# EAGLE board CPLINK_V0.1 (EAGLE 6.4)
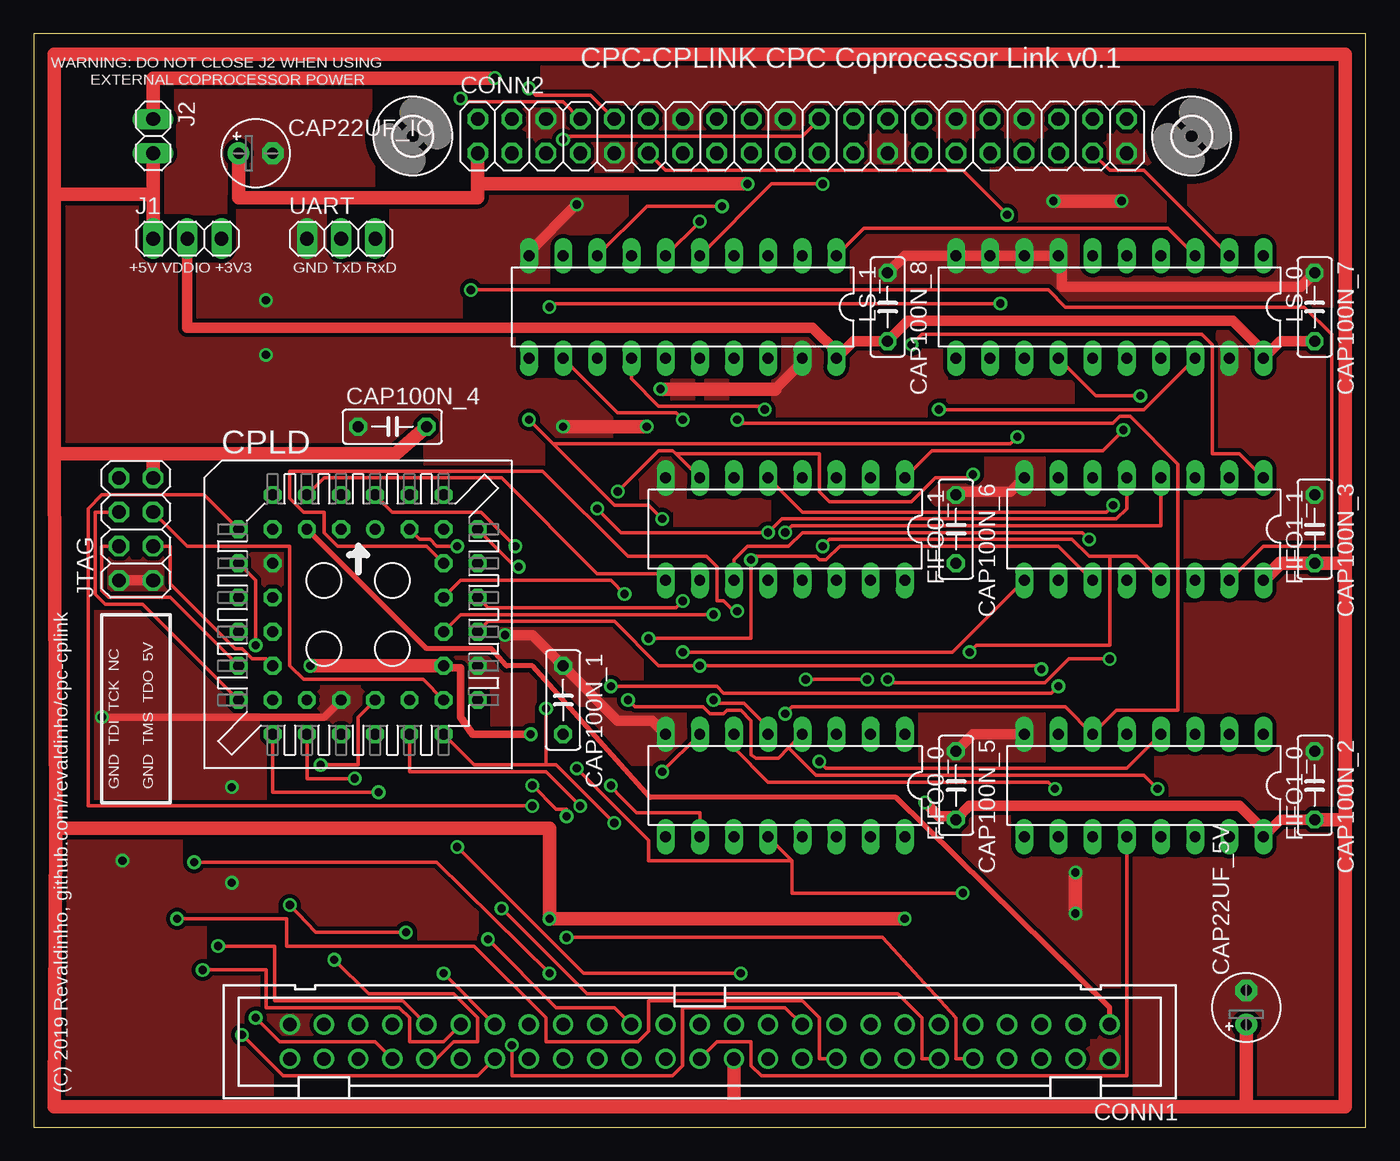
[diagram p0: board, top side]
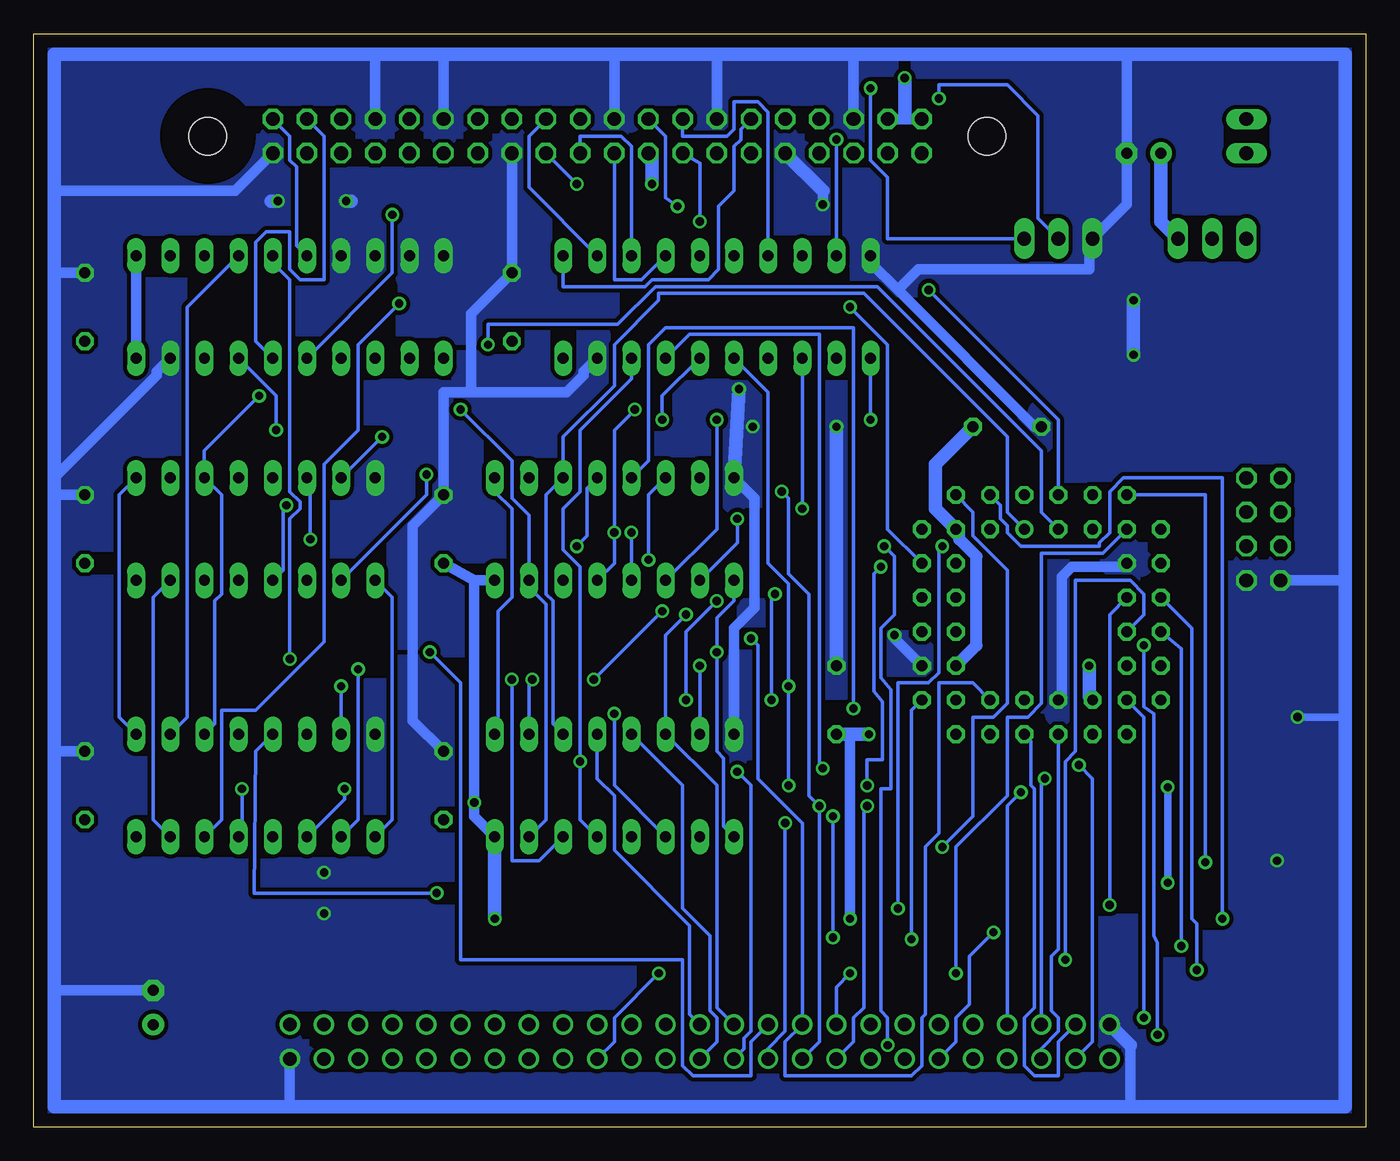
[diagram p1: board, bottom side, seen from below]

Size 99.06 x 81.28 mm. Coordinates in mm from the lower left corner, seen from the top.
Outline: 0,0 99.06,0 99.06,81.28 0,81.28 0,0
Copper layers (1*16): Top 0.035mm / dielectric 1.5mm / Bottom 0.035mm
Design rules "default": minimum track width 10mil, minimum drill 24mil, track to track 8mil, track to pad 8mil, pad to pad 8mil, via to via 8mil, smd to smd 8mil, copper to edge 40mil, drill to drill 8mil, minimum pad ring 10mil, minimum via ring 8mil, stop-mask expansion 4mil, vias tented up to drill 0mil, thermal gap 10mil
Net classes: 0 signal: width 0.254 mm, clearance 0.254 mm; 1 supply: width 0.559 mm, clearance 0.305 mm

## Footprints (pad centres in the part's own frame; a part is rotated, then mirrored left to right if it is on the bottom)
E2,5-5 = drill 0.813 pad 1.6: + -1.27,0 | drill 0.813 pad 1.6 octagon: - 1.27,0
C050-025X075 = drill 0.813 octagon: 1 -2.54,0; 2 2.54,0
PAK100/2500-50 = drill 1 pad 1.422: 1 -30.48,-1.27; 2 -30.48,1.27; 3 -27.94,-1.27; 4 -27.94,1.27; 5 -25.4,-1.27; 6 -25.4,1.27; 7 -22.86,-1.27; 8 -22.86,1.27; 9 -20.32,-1.27; 10 -20.32,1.27; 11 -17.78,-1.27; 12 -17.78,1.27; 13 -15.24,-1.27; 14 -15.24,1.27; 15 -12.7,-1.27; 16 -12.7,1.27; 17 -10.16,-1.27; 18 -10.16,1.27; 19 -7.62,-1.27; 20 -7.62,1.27; 21 -5.08,-1.27; 22 -5.08,1.27; 23 -2.54,-1.27; 24 -2.54,1.27; 25 0,-1.27; 26 0,1.27; 27 2.54,-1.27; 28 2.54,1.27; 29 5.08,-1.27; 30 5.08,1.27; 31 7.62,-1.27; 32 7.62,1.27; 33 10.16,-1.27; 34 10.16,1.27; 35 12.7,-1.27; 36 12.7,1.27; 37 15.24,-1.27; 38 15.24,1.27; 39 17.78,-1.27; 40 17.78,1.27; 41 20.32,-1.27; 42 20.32,1.27; 43 22.86,-1.27; 44 22.86,1.27; 45 25.4,-1.27; 46 25.4,1.27; 47 27.94,-1.27; 48 27.94,1.27; 49 30.48,-1.27; 50 30.48,1.27
2X20 = drill 1.016 octagon: 1 -24.13,-1.27; 2 -24.13,1.27; 3 -21.59,-1.27; 4 -21.59,1.27; 5 -19.05,-1.27; 6 -19.05,1.27; 7 -16.51,-1.27; 8 -16.51,1.27; 9 -13.97,-1.27; 10 -13.97,1.27; 11 -11.43,-1.27; 12 -11.43,1.27; 13 -8.89,-1.27; 14 -8.89,1.27; 15 -6.35,-1.27; 16 -6.35,1.27; 17 -3.81,-1.27; 18 -3.81,1.27; 19 -1.27,-1.27; 20 -1.27,1.27; 21 1.27,-1.27; 22 1.27,1.27; 23 3.81,-1.27; 24 3.81,1.27; 25 6.35,-1.27; 26 6.35,1.27; 27 8.89,-1.27; 28 8.89,1.27; 29 11.43,-1.27; 30 11.43,1.27; 31 13.97,-1.27; 32 13.97,1.27; 33 16.51,-1.27; 34 16.51,1.27; 35 19.05,-1.27; 36 19.05,1.27; 37 21.59,-1.27; 38 21.59,1.27; 39 24.13,-1.27; 40 24.13,1.27
PLCC-S44-SOCKET = drill 0.813: 1 1.27,6.35 | drill 0.813 octagon: 2 -1.27,8.89; 3 -1.27,6.35; 4 -3.81,8.89; 5 -3.81,6.35; 6 -6.35,8.89; 7 -8.89,6.35; 8 -6.35,6.35; 9 -8.89,3.81; 10 -6.35,3.81; 11 -8.89,1.27; 12 -6.35,1.27; 13 -8.89,-1.27; 14 -6.35,-1.27; 15 -8.89,-3.81; 16 -6.35,-3.81; 17 -8.89,-6.35; 18 -6.35,-8.89; 19 -6.35,-6.35; 20 -3.81,-8.89; 21 -3.81,-6.35; 22 -1.27,-8.89; 23 -1.27,-6.35; 24 1.27,-8.89; 25 1.27,-6.35; 26 3.81,-8.89; 27 3.81,-6.35; 28 6.35,-8.89; 29 8.89,-6.35; 30 6.35,-6.35; 31 8.89,-3.81; 32 6.35,-3.81; 33 8.89,-1.27; 34 6.35,-1.27; 35 8.89,1.27; 36 6.35,1.27; 37 8.89,3.81; 38 6.35,3.81; 39 8.89,6.35; 40 6.35,8.89; 41 6.35,6.35; 42 3.81,8.89; 43 3.81,6.35; 44 1.27,8.89
DIL16 = drill 0.813 long: 1 -8.89,-3.81; 2 -6.35,-3.81; 3 -3.81,-3.81; 4 -1.27,-3.81; 5 1.27,-3.81; 6 3.81,-3.81; 7 6.35,-3.81; 8 8.89,-3.81; 9 8.89,3.81; 10 6.35,3.81; 11 3.81,3.81; 12 1.27,3.81; 13 -1.27,3.81; 14 -3.81,3.81; 15 -6.35,3.81; 16 -8.89,3.81
2,8 = hole 2.8: 0,0
1X03 = drill 1.016 long: 1 -2.54,0; 2 0,0; 3 2.54,0
1X02 = drill 1.016 long: 1 -1.27,0; 2 1.27,0
2X04 = drill 1.016 octagon: 1 -3.81,-1.27; 2 -3.81,1.27; 3 -1.27,-1.27; 4 -1.27,1.27; 5 1.27,-1.27; 6 1.27,1.27; 7 3.81,-1.27; 8 3.81,1.27
DIL20 = drill 0.813 long: 1 -11.43,-3.81; 2 -8.89,-3.81; 3 -6.35,-3.81; 4 -3.81,-3.81; 5 -1.27,-3.81; 6 1.27,-3.81; 7 3.81,-3.81; 8 6.35,-3.81; 9 8.89,-3.81; 10 11.43,-3.81; 11 11.43,3.81; 12 8.89,3.81; 13 6.35,3.81; 14 3.81,3.81; 15 1.27,3.81; 16 -1.27,3.81; 17 -3.81,3.81; 18 -6.35,3.81; 19 -8.89,3.81; 20 -11.43,3.81

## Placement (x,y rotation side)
CAP22UF_5V  [E2,5-5]  90.17,8.89 90 top
CAP22UF_IO  [E2,5-5]  16.51,72.39 0 top
CAP100N_1  [C050-025X075]  39.37,31.75 270 top
CAP100N_2  [C050-025X075]  95.25,25.4 270 top
CAP100N_3  [C050-025X075]  95.25,44.45 270 top
CAP100N_4  [C050-025X075]  26.67,52.07 0 top
CAP100N_5  [C050-025X075]  68.58,25.4 270 top
CAP100N_6  [C050-025X075]  68.58,44.45 270 top
CAP100N_7  [C050-025X075]  95.25,60.96 270 top
CAP100N_8  [C050-025X075]  63.5,60.96 270 top
CONN1  [PAK100/2500-50]  49.53,6.35 180 top
CONN2  [2X20]  57.15,73.66 0 top
CPLD  [PLCC-S44-SOCKET]  24.13,38.1 0 top
FIFO0_0  [DIL16]  55.88,25.4 180 top
FIFO0_1  [DIL16]  55.88,44.45 180 top
FIFO1_0  [DIL16]  82.55,25.4 180 top
FIFO1_1  [DIL16]  82.55,44.45 180 top
H1  [2,8]  86.11,73.66 0 top
H2  [2,8]  28.19,73.66 0 top
J1  [1X03]  11.43,66.04 0 top
J2  [1X02]  8.89,73.66 270 top
JTAG  [2X04]  7.62,44.45 90 top
LS_0  [DIL20]  80.01,60.96 180 top
LS_1  [DIL20]  48.26,60.96 180 top
UART  [1X03]  22.86,66.04 0 top

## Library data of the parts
CAP22UF_5V CAP22UF_IO CAP100N_1-CAP100N_8 = resistor
CONN1 = con-3m
CONN2 J1 J2 JTAG UART = pinhead
CPLD FIFO0_0 FIFO0_1 FIFO1_0 FIFO1_1 LS_0 LS_1 = ic-package
H1 H2 = holes

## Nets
A0: CONN1.33 CPLD.6
A1: CONN1.34 CPLD.7
A2: CONN1.35
A3: CONN1.36
A4: CONN1.37 CPLD.8
A5: CONN1.38 CPLD.9
A6: CONN1.39 CPLD.11
A7: CONN1.40 CPLD.12
A8: CONN1.41 CPLD.13
A9: CONN1.42 CPLD.14
A10: CONN1.43 CPLD.18
A11: CONN1.44 CPLD.19
A12: CONN1.45 CPLD.20
A13: CONN1.46 CPLD.22
A14: CONN1.47 CPLD.24
A15: CONN1.48 CPLD.25
BUSACK_B: CONN1.13
BUSRESET_B: CONN1.11
BUSRQ_B: CONN1.14
CLK: CONN1.1 CPLD.5
CURSOR: CONN1.5
D0: CONN1.25 CPLD.36 FIFO0_0.4 FIFO1_0.13
D1: CONN1.26 CPLD.35 FIFO0_0.5 FIFO1_0.12
D2: CONN1.27 CPLD.34 FIFO0_0.6 FIFO1_0.11
D3: CONN1.28 CPLD.33 FIFO0_0.7 FIFO1_0.10
D4: CONN1.29 CPLD.29 FIFO0_1.4 FIFO1_1.13
D5: CONN1.30 CPLD.28 FIFO0_1.5 FIFO1_1.12
D6: CONN1.31 CPLD.27 FIFO0_1.6 FIFO1_1.11
D7: CONN1.32 CPLD.26 FIFO0_1.7 FIFO1_1.10
EXP_B: CONN1.3
FIFO_HOST_DIR: CPLD.38 FIFO0_0.2
FIFO_HOST_DOR: CPLD.37 FIFO1_0.14
FIFO_SLAVE_DIR: FIFO1_0.2 LS_0.4
FIFO_SLAVE_DOR: FIFO0_0.14 LS_0.5
HALT_B: CONN1.17
HOST_FIFO_OEB: CPLD.3 FIFO1_0.1 FIFO1_1.1
HOST_FIFO_RESET: CPLD.4 FIFO0_0.9 FIFO0_1.9 FIFO1_0.9 FIFO1_1.9
HOST_FIFO_SI: CPLD.1 FIFO0_0.3 FIFO0_1.3
HOST_FIFO_SOB: CPLD.2 FIFO1_0.15 FIFO1_1.15
INT_B: CONN1.16
IOREQ_B: CONN1.20 CPLD.40
LPEN: CONN1.4
M1_B: CONN1.22
MREQ_B: CONN1.23
NMI_B: CONN1.15
PI_GPIO_02: CONN2.3
PI_GPIO_03: CONN2.5
PI_GPIO_04: CONN2.7
PI_GPIO_05: CONN2.29
PI_GPIO_06: CONN2.31
PI_GPIO_07: CONN2.26
PI_GPIO_08: CONN2.24 LS_1.2
PI_GPIO_09: CONN2.21 LS_1.3
PI_GPIO_10: CONN2.19 LS_1.4
PI_GPIO_11: CONN2.23 LS_1.5
PI_GPIO_12: CONN2.32
PI_GPIO_13: CONN2.33
PI_GPIO_14: CONN2.8 UART.2
PI_GPIO_15: CONN2.10 UART.3
PI_GPIO_16: CONN2.36
PI_GPIO_17: CONN2.11 LS_0.15
PI_GPIO_18: CONN2.12 LS_0.3 LS_1.1
PI_GPIO_19: CONN2.35
PI_GPIO_20: CONN2.38 LS_0.16
PI_GPIO_21: CONN2.40 LS_0.6
PI_GPIO_22: CONN2.15 LS_1.6
PI_GPIO_23: CONN2.16 LS_1.7
PI_GPIO_24: CONN2.18 LS_1.8
PI_GPIO_25: CONN2.22 LS_1.9
PI_GPIO_26: CONN2.37 LS_0.2
PI_GPIO_27: CONN2.13
RAMDIS: CONN1.6
RAMRD_B: CONN1.7
RD_B: CONN1.19 CPLD.44
READY: CONN1.12 CPLD.43
RESET_B: CONN1.10 CPLD.39
RFSH_B: CONN1.21
ROMDIS: CONN1.8
ROMEN_B: CONN1.9
SCL: CONN2.28
SD0: FIFO0_0.13 FIFO1_0.4 LS_1.18
SD1: FIFO0_0.12 FIFO1_0.5 LS_1.17
SD2: FIFO0_0.11 FIFO1_0.6 LS_1.16
SD3: FIFO0_0.10 FIFO1_0.7 LS_1.15
SD4: FIFO0_1.13 FIFO1_1.4 LS_1.14
SD5: FIFO0_1.12 FIFO1_1.5 LS_1.13
SD6: FIFO0_1.11 FIFO1_1.6 LS_1.12
SD7: FIFO0_1.10 FIFO1_1.7 LS_1.11
SDA: CONN2.27
SLAVE_FIFO_SI: FIFO1_0.3 FIFO1_1.3 LS_0.14
SLAVE_FIFO_SOB: FIFO0_0.15 FIFO0_1.15 LS_0.18
SLAVE_FIFO_WNR: FIFO0_0.1 FIFO0_1.1 LS_0.17
SOUND: CONN1.50
TCK: CPLD.17 JTAG.6
TDI: CPLD.15 JTAG.4
TDO: CPLD.30 JTAG.5
TMS: CPLD.16 JTAG.3
VDD [supply]: CAP22UF_5V.+ CAP100N_1.2 CAP100N_2.2 CAP100N_3.2 CAP100N_4.2 CAP100N_5.2 CAP100N_6.2 CONN1.24 CPLD.21 CPLD.32 CPLD.41 FIFO0_0.16 FIFO0_1.16 FIFO1_0.16 FIFO1_1.16 J1.1 J2.2 JTAG.7
VDD_3V3 [supply]: CAP22UF_IO.+ CONN2.1 CONN2.17 J1.3
VDD_IO [supply]: CAP100N_7.2 CAP100N_8.2 J1.2 LS_0.1 LS_0.20 LS_1.20
VDD_PI [supply]: CONN2.2 CONN2.4 J2.1
VSS [supply]: CAP22UF_5V.- CAP22UF_IO.- CAP100N_1.1 CAP100N_2.1 CAP100N_3.1 CAP100N_4.1 CAP100N_5.1 CAP100N_6.1 CAP100N_7.1 CAP100N_8.1 CONN1.2 CONN1.49 CONN2.6 CONN2.9 CONN2.14 CONN2.20 CONN2.25 CONN2.30 CONN2.34 CONN2.39 CPLD.10 CPLD.23 CPLD.31 FIFO0_0.8 FIFO0_1.8 FIFO1_0.8 FIFO1_1.8 JTAG.1 JTAG.2 LS_0.7 LS_0.8 LS_0.9 LS_0.10 LS_0.19 LS_1.10 LS_1.19 UART.1
WR_B: CONN1.18 CPLD.42

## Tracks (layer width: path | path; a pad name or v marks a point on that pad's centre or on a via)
A0  (via drill 0.61)
  Top 0.254: v11.94,19.68 29.97,19.68 v38.35,11.43
  Bottom 0.254: CPLD.6 11.94,46.99 v11.94,19.68 | v38.35,11.43 39.37,10.41 CONN1.33
A1  (via drill 0.61)
  Top 0.254: CPLD.7 12.7,46.99 5.08,46.99 4.06,45.97 4.06,23.88 v37.08,23.88
  Bottom 0.254: v37.08,23.88 37.34,23.62 37.34,8.89 38.1,8.13 38.1,6.35 CONN1.34
A4  (via drill 0.61)
  Top 0.254: CONN1.37 v30.48,11.43
  Bottom 0.254: CPLD.8 19.56,42.67 24.13,42.67 24.13,31.5 25.15,30.48 26.67,30.48 26.67,24.64 30.48,20.83 v30.48,11.43
A5  (via drill 0.61)
  Top 0.254: CPLD.9 16.51,40.64 v16.51,35.81 | v15.49,6.86 18.54,3.81 33.02,3.81 CONN1.38
  Bottom 0.254: v16.51,35.81 16.51,31.24 15.75,30.73 15.75,14.22 15.49,13.72 v15.49,6.86
A6  (via drill 0.61)
  Top 0.254: v12.57,11.68 17.27,11.68 17.27,8.89 27.18,8.89 27.94,8.13 27.94,6.35 30.48,6.35 CONN1.39
  Bottom 0.254: CPLD.11 12.95,37.08 12.95,15.49 12.57,15.11 v12.57,11.68
A7  (via drill 0.61)
  Top 0.254: v27.69,14.48 20.95,14.48 19.68,15.88 v19.05,16.51
  Bottom 0.254: CPLD.12 19.05,38.1 v19.05,16.51 | v27.69,14.48 29.46,12.7 29.46,9.14 30.48,8.13 30.48,6.35 CONN1.40
A8  (via drill 0.61)
  Top 0.254: v13.72,13.46 17.91,13.46 17.91,9.4 27.43,9.4 CONN1.41
  Bottom 0.254: CPLD.13 13.72,35.56 v13.72,13.46
A9  (via drill 0.61)
  Top 0.254: v22.35,12.45 24.89,9.91 31.24,9.91 33.02,8.13 33.02,6.35 31.24,6.35 29.97,5.08 CONN1.42
  Bottom 0.254: CPLD.14 16.51,38.1 16.51,39.62 17.53,40.64 21.59,40.64 21.59,27.94 22.35,27.18 v22.35,12.45
A10  (via drill 0.61)
  Top 0.254: CPLD.18 17.78,24.89 v25.65,24.89
  Bottom 0.254: v25.65,24.89 26.67,23.88 CONN1.43
A11  (via drill 0.61)
  Top 0.254: v16.51,8.13 18.29,6.35 25.4,6.35 CONN1.44
  Bottom 0.254: CPLD.19 16.51,30.48 v16.51,8.13
A12  (via drill 0.61)
  Top 0.254: CPLD.20 20.32,25.91 v23.88,25.91
  Bottom 0.254: v23.88,25.91 24.13,25.65 CONN1.45
A13
  Bottom 0.254: CPLD.22 22.86,13.21 23.37,12.7 23.37,8.64 22.86,8.13 22.86,7.11 24.13,5.84 CONN1.46
A14
  Bottom 0.254: CPLD.24 24.89,28.7 24.89,25.4 24.64,25.15 24.64,8.89 25.4,8.13 25.4,4.57 24.64,3.81 22.86,3.81 22.86,6.35 CONN1.47
A15  (via drill 0.61)
  Top 0.254: CPLD.25 24.13,30.48 24.13,26.92 v21.34,26.92
  Bottom 0.254: v21.34,26.92 20.32,25.91 20.32,6.35 CONN1.48
CLK
  Top 0.381: CPLD.5 29.21,35.56 34.04,35.56 35.18,34.29 37.08,34.29 45.85,24.51 64.14,24.51 80.01,8.89 CONN1.1
D0  (via drill 0.61)
  Top 0.254: CPLD.36 31.75,40.64 42.93,40.64 v43.94,39.62 | v44.2,31.75 44.7,31.24 49.78,31.24 50.29,30.73 51.31,30.73 51.56,30.99 52.58,30.99 53.34,30.23 53.34,27.69 53.72,27.43 55.37,27.43 56.13,28.19 | FIFO0_0.4 56.13,28.19 | v83.57,25.15 82.55,26.16 58.17,26.16 56.13,28.19
  Bottom 0.254: v43.94,39.62 44.2,39.37 v44.2,31.75 | FIFO1_0.13 83.57,21.84 v83.57,25.15 | CONN1.25 50.29,8.38 50.29,14.99 55.88,20.57 55.88,24.64 57.15,25.91 FIFO0_0.4
D1  (via drill 0.61)
  Top 0.254: FIFO1_0.12 81.28,3.81 54.1,3.81 53.34,4.57 53.34,6.35 50.8,6.35 CONN1.26 | CPLD.35 33.78,38.61 47.75,38.61 v48.26,39.12 | v50.55,31.75 50.8,31.5 52.83,31.5 54.61,29.72 FIFO0_0.5
  Bottom 0.254: FIFO0_0.5 50.8,25.4 50.8,16.26 48.77,14.22 48.77,8.64 48.26,8.13 48.26,6.35 CONN1.26 | v48.26,39.12 50.55,36.83 v50.55,31.75
D2  (via drill 0.61)
  Top 0.254: CPLD.34 31.75,38.1 v50.55,38.1 | v75.95,25.15 75.44,25.65 54.61,25.65 52.07,28.19 FIFO0_0.6
  Bottom 0.254: v50.55,38.1 52.07,36.58 FIFO0_0.6 48.26,25.4 48.26,8.89 CONN1.27 | FIFO1_0.11 75.95,24.38 v75.95,25.15
D3  (via drill 0.61)
  Top 0.254: CPLD.33 33.78,37.59 43.18,37.59 46.48,34.29 v49.53,34.29 74.68,34.29 v74.93,34.04 | FIFO0_0.7 v46.74,26.42
  Bottom 0.254: FIFO0_0.7 v49.53,34.29 | FIFO1_0.10 74.93,22.86 v74.93,34.04 | CONN1.28 46.23,5.84 46.23,6.6 45.72,7.11 45.72,25.4 v46.74,26.42
D4  (via drill 0.61)
  Top 0.254: v58.67,43.18 59.18,43.69 77.22,43.69 78.49,42.42 80.01,42.42 | 80.01,42.42 82.04,42.42 FIFO1_1.13 | v33.78,13.97 38.86,8.89 43.18,8.89 CONN1.29 | 80.01,42.42 80.01,35.81 70.1,35.81 v69.6,35.31
  Bottom 0.254: FIFO0_1.4 57.91,47.5 57.91,43.94 v58.67,43.18 | CPLD.29 33.78,30.99 v33.78,13.97 | v69.6,35.31 67.31,33.02 67.31,12.45 50.8,12.45 50.8,4.57 50.04,3.81 45.72,3.81 45.72,6.35 CONN1.29
D5  (via drill 0.61)
  Top 0.254: v80.26,46.23 79.76,45.72 57.15,45.72 FIFO0_1.5 | CPLD.28 32.77,26.92 38.1,26.92 | 38.1,26.92 38.86,26.92 v43.18,22.61 | 38.1,26.92 v38.1,31.11
  Bottom 0.254: FIFO1_1.12 80.52,41.4 80.52,45.97 v80.26,46.23 | v43.18,22.61 43.18,7.11 44.45,5.84 CONN1.30 | FIFO0_1.5 53.34,49.53 53.34,58.17 52.07,59.44 38.1,59.44 v38.1,31.11
D6  (via drill 0.61)
  Top 0.254: FIFO1_1.11 76.2,43.18 59.94,43.18 58.93,42.16 58.42,42.16 58.17,42.42 53.59,42.42 v53.34,42.16 53.34,36.32 v45.72,36.32
  Bottom 0.254: FIFO0_1.6 53.34,46.99 v53.34,42.16 | CPLD.27 29.21,33.02 31.75,33.02 31.75,21.84 32.77,20.83 32.77,8.38 33.02,8.13 33.02,4.57 33.78,3.81 43.18,3.81 43.18,6.35 CONN1.31 41.91,22.61 45.21,25.91 45.21,35.81 v45.72,36.32
D7  (via drill 0.61)
  Top 0.254: CPLD.26 27.94,26.42 38.1,26.42 v40.64,23.88 | 47.75,50.04 47.5,50.29 46.48,50.29 v43.43,47.24 | 47.75,50.04 FIFO0_1.7 | v69.85,48.51 69.6,48.26 67.06,48.26 65.28,46.48 59.18,46.48 58.42,47.24 58.42,50.04 47.75,50.04
  Bottom 0.254: CONN1.32 40.64,6.35 v40.64,23.88 41.4,24.64 41.4,39.62 42.93,41.15 42.93,46.74 v43.43,47.24 | FIFO1_1.10 69.85,46.99 v69.85,48.51
FIFO_HOST_DIR  (via drill 0.61)
  Top 0.254: CPLD.38 29.21,43.18 22.61,43.18 21.59,44.2 21.59,45.72 20.07,45.72 19.05,46.74 19.05,48.77 37.85,48.77 44.2,42.42 50.04,42.42 50.8,41.66 50.8,39.12 51.31,39.12 52.07,38.35 v52.32,38.35 | v61.98,33.27 v57.4,33.27
  Bottom 0.254: v57.4,33.27 v52.32,38.35 | v61.98,33.27 62.23,33.02 FIFO0_0.2
FIFO_HOST_DOR  (via drill 0.61)
  Top 0.254: v38.35,60.96 38.61,61.21 v71.88,61.21
  Bottom 0.254: CPLD.37 35.56,44.45 35.56,58.17 v38.35,60.96 | v71.88,61.21 74.93,58.17 74.93,51.82 77.47,49.28 77.47,36.07 82.55,30.99 85.09,30.99 85.09,22.86 FIFO1_0.14
FIFO_SLAVE_DIR
  Bottom 0.254: FIFO1_0.2 87.63,30.48 87.63,60.96 LS_0.4
FIFO_SLAVE_DOR  (via drill 0.61)
  Top 0.254: v63.5,33.27 63.75,33.02 75.18,33.02 76.96,34.8 v80.01,34.8
  Bottom 0.254: FIFO0_0.14 61.47,19.81 63.5,19.81 v63.5,33.27 | v80.01,34.8 80.01,45.21 79.25,45.97 79.25,46.48 80.01,47.24 80.01,62.99 81.28,64.26 LS_0.5
HOST_FIFO_OEB  (via drill 0.61)
  Top 0.254: v65.28,58.17 66.04,58.93 86.87,58.93 87.63,58.17 87.63,50.04 89.66,50.04 FIFO1_1.1
  Bottom 0.254: CPLD.3 24.13,45.72 24.13,50.29 36.32,62.48 52.83,62.48 55.63,59.69 65.28,59.69 v65.28,58.17 | FIFO1_0.1 92.71,30.48 92.71,46.99 FIFO1_1.1
HOST_FIFO_RESET  (via drill 0.61)
  Top 0.254: CPLD.4 21.59,48.26 34.8,48.26 41.91,41.15 46.48,41.15 FIFO0_1.9 | FIFO1_1.9 68.33,35.31 v48.26,35.31
  Bottom 0.254: FIFO1_0.9 72.39,22.86 72.39,39.37 FIFO1_1.9 | FIFO0_0.9 47.75,22.35 47.75,27.43 48.26,27.94 v48.26,35.31 48.26,37.85 46.99,39.12 FIFO0_1.9
HOST_FIFO_SI
  Bottom 0.254: CPLD.1 26.67,45.72 26.67,51.31 37.34,61.98 52.58,61.98 52.58,61.47 55.88,58.17 55.88,55.12 59.69,51.31 FIFO0_1.3 60.96,46.99 60.96,39.62 60.45,39.12 60.45,29.97 FIFO0_0.3
HOST_FIFO_SOB  (via drill 0.61)
  Top 0.254: v32.51,62.23 75.44,62.23 76.71,60.96 94.49,60.96 96.52,58.93 96.52,43.18 91.44,43.18 FIFO1_1.15
  Bottom 0.254: FIFO1_0.15 90.17,22.86 90.17,39.37 FIFO1_1.15 | CPLD.2 22.86,52.58 v32.51,62.23
IOREQ_B  (via drill 0.61)
  Top 0.254: v31.5,20.83 40.89,11.43 v52.58,11.43
  Bottom 0.254: CPLD.40 29.21,45.72 29.21,43.94 26.67,41.4 26.67,31.5 27.69,30.48 29.21,30.48 29.21,23.11 v31.5,20.83 | v52.58,11.43 55.88,8.13 55.88,6.35 CONN1.20
PI_GPIO_08
  Bottom 0.254: LS_1.2 62.23,69.85 62.23,73.66 CONN2.24
PI_GPIO_09
  Bottom 0.254: LS_1.3 54.61,72.9 55.37,73.66 58.42,73.66 CONN2.21
PI_GPIO_10
  Bottom 0.254: LS_1.4 53.85,62.99 55.88,62.99 CONN2.19
PI_GPIO_11  (via drill 0.61)
  Top 0.254: LS_1.5 54.86,70.1 v58.67,70.1
  Bottom 0.254: CONN2.23 v58.67,70.1
PI_GPIO_14  (via drill 0.61)
  Top 0.254: v31.75,76.45 32,76.2 39.37,76.2 CONN2.8
  Bottom 0.254: UART.2 24.38,67.56 24.38,75.18 26.67,77.47 31.75,77.47 v31.75,76.45
PI_GPIO_15  (via drill 0.61)
  Top 0.254: v36.83,77.22 37.34,76.71 41.4,76.71 CONN2.10
  Bottom 0.254: UART.3 35.56,66.04 35.56,70.61 36.83,71.88 v36.83,77.22
PI_GPIO_17  (via drill 0.61)
  Top 0.254: v72.39,67.82 69.09,71.12 46.99,71.12 CONN2.11
  Bottom 0.254: LS_0.15 72.39,63.5 v72.39,67.82
PI_GPIO_18
  Top 0.254: LS_1.1 61.72,66.8 84.33,66.8 LS_0.3
  Bottom 0.254: CONN2.12 46.48,74.17 46.48,73.41 46.99,72.9 46.99,69.6 48.13,68.45 48.13,63.75 48.9,62.99 53.09,62.99 53.59,62.48 59.69,62.48 LS_1.1
PI_GPIO_20
  Bottom 0.254: LS_0.16 82.55,58.42 82.55,65.79 81.79,66.55 80.01,66.55 80.01,63.75 79.25,62.99 77.47,62.99 77.47,73.66 CONN2.38
PI_GPIO_21
  Bottom 0.254: LS_0.6 79.5,65.53 79.5,71.37 80.01,71.88 80.01,73.66 CONN2.40
PI_GPIO_22  (via drill 0.61)
  Top 0.254: v49.53,67.31 LS_1.6
  Bottom 0.254: v49.53,67.31 49.53,71.63 CONN2.15
PI_GPIO_23
  Bottom 0.254: LS_1.7 44.45,75.44 45.21,76.2 46.99,76.2 46.99,74.17 47.5,73.66 50.8,73.66 CONN2.16
PI_GPIO_24  (via drill 0.61)
  Top 0.254: LS_1.8 45.59,68.45 v51.18,68.45
  Bottom 0.254: v51.18,68.45 52.07,69.09 52.07,73.66 CONN2.18
PI_GPIO_25  (via drill 0.61)
  Top 0.254: v39.37,73.41 39.62,73.66 57.15,73.66 CONN2.22
  Bottom 0.254: v39.37,73.41 LS_1.9
PI_GPIO_26
  Top 0.254: LS_0.2 82.55,71.12 80.01,71.12 CONN2.37
RD_B  (via drill 0.61)
  Top 0.254: CPLD.44 26.67,45.72 33.27,45.72 v35.81,43.18 | v35.56,6.1 35.56,3.81 47.5,3.81 48.26,4.57 48.26,8.89 55.88,8.89 CONN1.19
  Bottom 0.254: v35.81,43.18 35.05,42.42 35.05,38.1 36.07,37.08 36.07,33.4 35.31,32.51 35.31,25.15 36.07,25.15 36.07,8.64 35.56,8.13 v35.56,6.1
READY  (via drill 0.61)
  Top 0.254: CPLD.43 28.7,43.69 29.46,43.69 29.97,43.18 v31.5,43.18 | v34.8,16.26 41.15,9.91 64.26,9.91 66.04,8.13 66.04,5.08 CONN1.12
  Bottom 0.254: v31.5,43.18 31.75,42.93 31.75,33.78 32.51,33.02 34.8,33.02 v34.8,16.26
RESET_B  (via drill 0.61)
  Top 0.254: CPLD.39 35.81,41.66 v36.07,41.66 | v37.08,25.4 38.86,23.62 39.62,23.62 v39.62,23.11 | v39.62,14.1 63.12,14.1 68.58,8.13 68.58,5.08 CONN1.10
  Bottom 0.254: v36.07,41.66 36.58,41.15 36.58,32.38 35.94,31.62 35.94,27.3 37.08,27.3 v37.08,25.4 | v39.62,14.1 v39.62,23.11
SD0  (via drill 0.61)
  Top 0.254: FIFO1_0.4 81.28,26.67 58.93,26.67 v58.42,27.18
  Bottom 0.254: FIFO0_0.13 58.42,22.86 v58.42,27.18 58.42,41.66 59.69,42.93 59.69,45.97 58.42,47.24 58.42,51.82 54.61,55.63 LS_1.18
SD1  (via drill 0.61)
  Top 0.254: 56.39,19.81 56.39,17.4 v69.09,17.4 | 56.39,19.81 FIFO0_0.12 | v40.39,26.67 45.72,21.34 45.72,19.81 56.39,19.81
  Bottom 0.254: v69.09,17.4 82.68,17.4 82.55,27.94 FIFO1_0.5 | LS_1.17 50.29,58.93 40.64,58.93 40.64,26.92 v40.39,26.67
SD2  (via drill 0.61)
  Top 0.254: v55.88,30.73 56.39,31.24 76.71,31.24 FIFO1_0.6 80.52,30.99 85.09,30.99 85.09,49.28 81.53,52.83 80.77,52.83 80.26,52.32 52.58,52.32 v52.32,52.58
  Bottom 0.254: FIFO0_0.11 55.88,25.4 v55.88,30.73 | LS_1.16 52.32,54.36 v52.32,52.58
SD3  (via drill 0.61)
  Top 0.254: FIFO0_0.10 49.53,23.37 44.83,23.37 43.43,24.77 v42.93,25.4 | v76.2,32.77 75.69,32.26 51.31,32.26 50.8,32.77 v42.93,32.77
  Bottom 0.254: v42.93,25.4 v42.93,32.77 42.93,40.39 44.45,41.91 44.45,54.61 LS_1.15 | v76.2,32.77 FIFO1_0.7
SD4  (via drill 0.61)
  Top 0.254: v54.36,53.34 54.1,53.59 46.48,53.59 44.45,55.63 LS_1.14 | FIFO1_1.4 83.82,44.7 56.39,44.7 v55.88,44.2
  Bottom 0.254: FIFO0_1.13 55.88,41.91 v55.88,44.2 55.88,51.82 v54.36,53.34
SD5  (via drill 0.61)
  Top 0.254: FIFO1_1.5 81.28,45.97 80.52,45.21 55.63,45.21 v54.61,44.2 43.69,44.2 v41.91,45.97
  Bottom 0.254: v54.61,44.2 FIFO0_1.12 | v41.91,45.97 LS_1.13
SD6  (via drill 0.61)
  Top 0.254: v48.26,52.58 47.75,53.09 43.43,53.09 LS_1.12 | v78.49,43.69 77.98,44.2 57.15,44.2 56.13,43.18 53.09,43.18 52.07,42.16 FIFO0_1.11
  Bottom 0.254: FIFO0_1.11 48.26,44.45 v48.26,52.58 | FIFO1_1.6 78.49,48.01 v78.49,43.69
SD7  (via drill 0.61)
  Top 0.254: v46.74,45.21 45.72,46.23 43.18,46.23 38.61,50.8 | v36.83,52.58 38.61,50.8 | v73.15,51.31 72.64,50.8 38.61,50.8
  Bottom 0.254: FIFO0_1.10 46.74,43.43 v46.74,45.21 | LS_1.11 v36.83,52.58 | v73.15,51.31 FIFO1_1.7
SLAVE_FIFO_SI  (via drill 0.61)
  Top 0.254: LS_0.14 78.99,54.36 v82.3,54.36
  Bottom 0.254: FIFO1_0.3 85.6,29.97 85.6,39.12 85.09,39.62 85.09,46.99 FIFO1_1.3 86.36,50.29 v82.3,54.36
SLAVE_FIFO_SOB  (via drill 0.61)
  Top 0.254: LS_0.18 82.55,53.34 v67.31,53.34
  Bottom 0.254: FIFO0_0.15 60.96,22.86 60.96,38.86 62.23,40.13 FIFO0_1.15 62.23,45.47 63.5,46.74 63.5,49.53 v67.31,53.34
SLAVE_FIFO_WNR  (via drill 0.61)
  Top 0.254: v81.03,51.82 79.5,50.29 66.8,50.29 FIFO0_1.1
  Bottom 0.254: FIFO0_0.1 64.52,29.46 64.52,38.35 63.5,39.37 63.5,45.97 64.77,47.24 FIFO0_1.1 | LS_0.17 81.03,54.36 v81.03,51.82
TCK
  Top 0.254: CPLD.17 8.13,38.86 5.33,38.86 4.57,39.62 4.57,45.72 JTAG.6
TDI
  Top 0.254: CPLD.15 10.16,39.37 5.59,39.37 5.08,39.88 5.08,43.18 JTAG.4
TDO
  Top 0.254: CPLD.30 28.96,33.27 20.07,33.27 19.05,34.29 19.05,43.18 11.43,43.18 JTAG.5
TMS
  Top 0.254: CPLD.16 17.27,34.8 16.26,34.8 15.49,35.56 14.99,35.56 10.16,40.39 10.16,43.18 JTAG.3
VDD  (via drill 0.61)
  Top 0.559: 30.61,34.16 31.75,34.16 31.75,30.48 32.64,29.21 v36.96,29.21 | 1.78,79.76 1.52,79.76
  Top 0.762: CAP100N_2.2 92.71,22.86 FIFO1_0.16 91.44,22.1 89.66,23.88 69.6,23.88 CAP100N_5.2 68.33,23.11 67.31,23.11 v66.29,24.13
  Top 1.016: 52.07,1.52 1.52,1.52 1.65,22.23 | 52.07,1.52 90.17,1.52 | 90.17,1.52 97.54,1.52 97.54,22.86 | 97.54,22.86 97.54,41.91 | 97.54,41.91 97.54,79.76 1.78,79.76 | 1.52,79.76 1.52,69.34 | 1.52,69.34 1.52,50.04 | 1.52,50.04 1.65,22.23 | CPLD.32 v20.57,34.29 | J2.2 8.89,69.34 | 8.89,69.34 J1.1 | FIFO1_1.16 92.71,41.91 CAP100N_3.2 97.54,41.91 | 1.65,22.23 38.35,22.23 v38.35,15.49 v64.77,15.49 | 52.07,1.52 CONN1.24 | 8.89,50.04 JTAG.7 | 1.52,50.04 8.89,50.04 | 90.17,1.52 CAP22UF_5V.+ | 1.52,69.34 8.89,69.34 | CAP100N_4.2 26.92,50.04 8.89,50.04 | 97.54,22.86 CAP100N_2.2
  Bottom 0.559: 38.35,29.21 CAP100N_1.2
  Bottom 0.762: FIFO0_0.16 66.29,23.11 v66.29,24.13 66.29,40.64 | FIFO0_1.16 66.29,40.64 | 66.29,40.64 CAP100N_6.2 | 20.57,32 CPLD.21 | 30.23,44.2 CPLD.41 | 38.35,29.21 v38.35,15.49
  Bottom 0.889: 30.23,44.2 30.23,43.69 28.96,42.42 28.96,35.81 CPLD.32
  Bottom 1.016: CPLD.41 32,45.97 32,49.28 CAP100N_4.2 | v20.57,34.29 20.57,32 | FIFO0_0.16 v64.77,15.49 | CAP100N_1.2 v36.96,29.21
VDD_3V3  (via drill 0.61)
  Top 1.016: 33.02,70.1 33.02,69.09 15.24,69.09 CAP22UF_IO.+ | 33.02,70.1 CONN2.1 | 33.02,70.1 v53.09,70.1
  Bottom 1.016: J1.3 15.24,67.31 CAP22UF_IO.+ | CONN2.17 53.09,72.14 v53.09,70.1
VDD_IO
  Top 0.762: CAP100N_7.2 92.71,58.42 LS_0.20 91.44,57.66 89.15,59.94 65.02,59.94 CAP100N_8.2 60.96,58.42 LS_1.20 59.69,57.66 57.91,59.44 11.43,59.44 J1.2
  Bottom 0.762: LS_0.20 LS_0.1
VDD_PI  (via drill 0.61)
  Top 1.016: J2.1 8.89,77.98 v34.29,77.98
  Bottom 0.559: 34.29,74.93 34.29,75.06
  Bottom 0.762: CONN2.2 34.29,74.93 CONN2.4
  Bottom 1.016: v34.29,77.98 34.29,75.06
VSS  (via drill 0.61)
  Top 0.559: CPLD.23 21.59,30.48 v5.08,30.48
  Top 0.762: FIFO0_0.8 45.97,30.23 43.43,30.23 CAP100N_1.1 37.08,36.58 v35.05,36.58 | CAP100N_8.1 64.77,64.77 LS_0.10 LS_0.9 LS_0.8 LS_0.7 76.45,64.52 76.45,62.48 94.23,62.48 CAP100N_7.1 | CAP100N_5.1 69.85,29.21 FIFO1_0.8 | CAP100N_6.1 68.83,47.24 72.64,47.24 FIFO1_1.8 | 55.12,54.86 57.15,56.9 LS_1.19 | v40.39,68.58 36.83,65.02 LS_1.10 | JTAG.1 JTAG.2
  Top 1.016: 55.12,54.86 v46.61,54.86 | v75.82,68.83 v80.9,68.83 | v77.47,18.92 v77.47,15.88 | v39.37,52.07 v45.59,52.07
  Bottom 0.559: 1.52,30.48 v5.08,30.48 | v14.73,25.27 v14.73,18.16
  Bottom 0.762: CPLD.23 22.61,32 22.61,40.89 21.84,41.66 17.78,41.66 CPLD.10 | CPLD.31 35.05,36.32 v35.05,36.58 | FIFO0_1.8 45.47,46.74 45.47,38.61 46.99,37.08 FIFO0_0.8 | CONN2.25 CAP100N_8.1 66.55,60.45 66.55,54.61 | LS_1.19 58.17,56.13 58.17,55.88 59.44,54.61 66.55,54.61 | 66.55,54.61 68.58,54.61 CAP100N_6.1 70.87,44.7 70.87,30.23 CAP100N_5.1 | CAP100N_4.1 24.64,52.07 34.8,62.23 | 34.8,62.23 36.83,64.26 LS_1.10 | v40.39,68.58 40.39,69.6 | 97.54,27.94 CAP100N_2.1 | 97.54,46.99 CAP100N_3.1 | LS_0.19 89.92,56.13 89.92,55.88 97.28,48.51 97.54,48.51 | 97.54,63.5 CAP100N_7.1 | 17.53,1.52 17.53,6.1 | 80.01,1.52 CONN1.2 | 38.1,79.76 CONN2.6 | 48.26,79.76 CONN2.14 | 55.88,79.76 CONN2.20 | 68.58,79.76 CONN2.30 | 73.66,79.76 CONN2.34 | CONN2.39 84.07,69.6 97.54,69.6 | 97.54,10.16 CAP22UF_5V.- | 1.52,40.64 JTAG.2 | 17.78,79.76 CAP22UF_IO.- 17.78,68.58 UART.1 20.57,65.79 20.57,63.75 33.27,63.75 34.8,62.23
  Bottom 1.016: v46.61,54.86 FIFO0_1.8 | 40.39,69.6 CONN2.9 | 17.53,6.1 CONN1.49 | 75.44,68.83 v75.82,68.83 | v80.9,68.83 81.41,68.83 | CAP100N_1.1 v39.37,52.07 | v17.27,61.47 v17.27,57.4 | 1.52,1.52 17.53,1.52 80.01,1.52 97.54,1.52 97.54,10.16 97.54,27.94 97.54,46.99 97.54,48.51 97.54,63.5 97.54,69.6 97.54,79.76 73.66,79.76 68.58,79.76 55.88,79.76 48.26,79.76 38.1,79.76 17.78,79.76 1.52,79.76 1.52,40.64 1.52,30.48 1.52,1.52
  other vias: 6.6,19.81
  pour Top: 0,0 0,81.28 99.06,81.28 99.06,0
  pour Bottom: 0,0 0,81.28 99.06,81.28 99.06,0
WR_B  (via drill 0.61)
  Top 0.254: v10.67,15.49 18.8,15.49 18.8,13.46 32.77,13.46 38.1,8.13 38.1,6.35 44.96,6.35 45.72,7.11 45.72,9.4 57.15,9.4 58.42,8.13 58.42,5.08 CONN1.18
  Bottom 0.254: CPLD.42 27.18,46.23 27.18,45.21 26.67,44.7 26.67,44.2 25.65,43.18 19.81,43.18 19.81,43.43 19.05,44.2 19.05,47.24 18.03,48.26 10.67,48.26 v10.67,15.49

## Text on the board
tPlace: WARNING: DO NOT CLOSE J2 WHEN USING | CPC-CPLINK CPC Coprocessor Link v0.1 | EXTERNAL COPROCESSOR POWER | +5V VDDIO +3V3 | GND TxD RxD | GND TDI TCK NC | GND TMS TDO 5V | (C) 2019 Revaldinho, github.com/revaldinho/cpc-cplink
